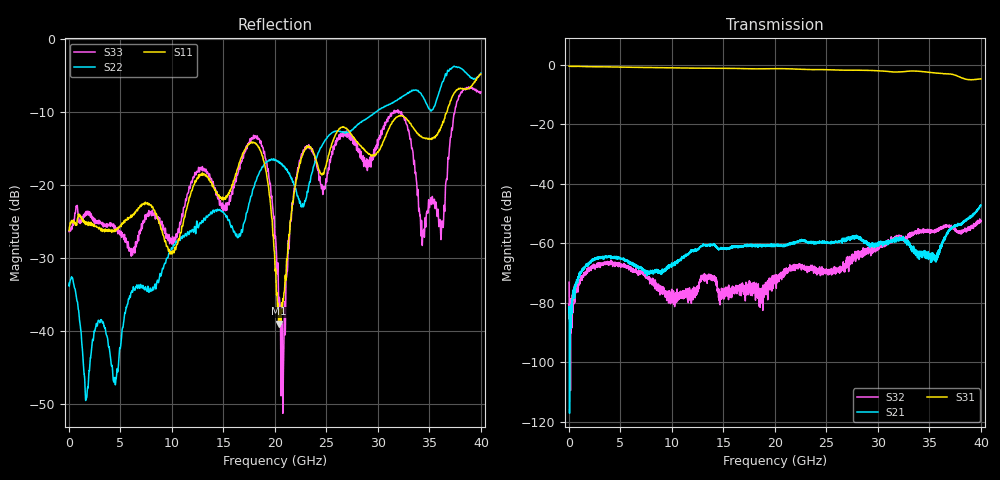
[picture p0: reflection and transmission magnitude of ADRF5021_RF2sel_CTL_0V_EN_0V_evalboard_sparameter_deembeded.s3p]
! Device:  ADRF5021
! Description: SOI MMIC SPDT Non-Reflective Switch
! Frequency:  9 kHz -  30 GHz
! Ports:
! 	RFC	= Port 1
!	RF1	= Port 2
!	RF2	= Port 3
! Vdd:  +3.3 Volt
! Vss:  -2.5 Volt
! Control:  0/+3.3 Volt
! State:  RF2 Selected (Vctl= 0 V, Ven= 0 V)
! Data:	Data was collected using a calibrated network analyzer with AFR software.
!	Fixtures were calculated using AFR and fixturing was applied to collect
!	this Deembedded  S Parameter data of ADRF5021.
! Note:	Analog Devices supplies this data as a sample of measured data at the package pin
!	for this product.  Your particular data for this product may vary.
!	Data was taken at 25 degrees C.
!	Analog Devices reserves the right to change this data at anytime.
# Hz S  dB  R 50
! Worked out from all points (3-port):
!   4000 points, 10 MHz to 40 GHz, reference 50 ohm
!   strongest paths, dB at 10 MHz, 10.01 GHz, 20.01 GHz, 30.01 GHz, 40 GHz:
!     S31: -0.6, -1.1, -1.4, -2.1, -4.8
!     S21: -83.4, -67.5, -60.9, -60.3, -47.2
!     S32: -73.1, -75.7, -71.4, -61.7, -52.5
!   lowest |S11| = -38.9 dB at 20.36 GHz (marker M1), VSWR 1.02, Z = 49 + j0.582 ohm
!   |S11| at or under -10 dB: start of sweep to 36.69 GHz
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1e7  -26.22 -0.6  -76.60 14.6  -0.55 -0.2
     -83.35 174.0  -33.42 -150.9  -80.22 -134.0
     -0.55 -0.2  -73.05 67.6  -26.38 -1.6
1.71e9  -25.12 -44.2  -67.35 61.7  -0.71 -21.3
        -67.45 60.4  -49.11 -65.2  -69.43 47.1
        -0.71 -21.3  -70.02 52.6  -24.08 -46.0
8.32e9  -23.48 -42.0  -69.17 77.6  -1.03 -100.7
        -68.87 79.9  -33.72 51.2  -73.68 -55.5
        -1.03 -100.7  -72.46 -61.1  -23.83 -36.9
1.795e10  -14.18 -121.9  -60.75 87.6  -1.44 143.5
          -60.70 88.2  -20.31 -88.6  -76.51 -44.8
          -1.44 143.6  -73.61 -52.1  -13.33 -138.3
2.001e10  -31.44 -157.2  -60.79 88.5  -1.40 117.9
          -60.91 85.6  -16.53 -20.2  -73.15 -65.3
          -1.39 118.0  -71.35 -65.6  -27.37 -111.4
2.036e10  -38.95 148.3  -60.93 88.1  -1.39 113.4
          -60.68 86.8  -16.75 -12.9  -70.61 -71.8
          -1.39 113.5  -71.38 -72.9  -36.49 -76.2
2.293e10  -15.15 -179.3  -59.04 77.8  -1.66 79.7
          -59.27 77.3  -22.18 -41.6  -68.38 -141.7
          -1.66 79.8  -68.23 -141.9  -14.78 165.7
2.917e10  -15.73 -89.4  -59.86 31.9  -1.99 -1.4
          -60.03 27.9  -10.67 -63.8  -62.60 135.4
          -1.98 -1.3  -61.31 138.1  -17.10 -113.7
3.616e10  -11.96 -109.4  -61.22 93.8  -3.01 -104.5
          -61.00 94.0  -6.35 -112.9  -54.69 2.2
          -3.01 -104.5  -54.63 1.9  -26.39 -170.7
4e10  -4.82 -122.8  -46.85 57.8  -4.84 -169.3
      -47.21 58.0  -4.69 -103.5  -52.65 -92.4
      -4.84 -169.1  -52.52 -90.2  -7.28 -69.9
